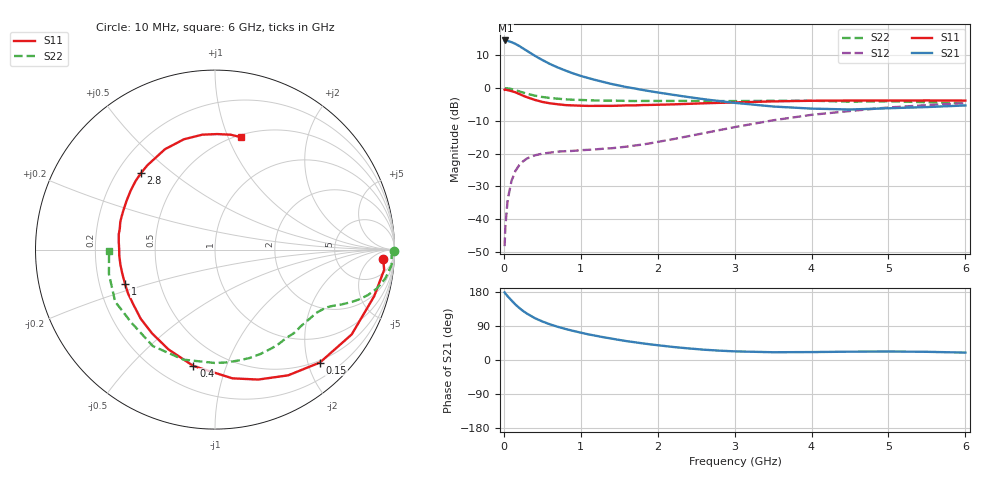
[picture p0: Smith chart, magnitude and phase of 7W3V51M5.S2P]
! Infineon Technologies  Discrete & RF Semiconductors
! BFS17W
! Si NPN RF Bipolar Junction Transistor in SOT323
! VCE = 3.5 V  IC = 1.5 mA
! Common Emitter S-Parameters:  August  1999
# GHz  S  MA  R  50
!  f  S11  S21  S12  S22
! GHz  MAG  ANG  MAG  ANG  MAG  ANG  MAG  ANG
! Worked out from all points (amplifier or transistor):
!   36 points, 10 MHz to 6 GHz, reference 50 ohm
!   highest |S21| = 14.5 dB at 20 MHz (marker M1)
!   |S21| within 3 dB of that: start of sweep to 288.9 MHz
!   unconditionally stable (mu >= 1): 905.5 MHz to end of sweep
!   at 250 MHz: K = 0.31, MSG = 17.2 dB, |S12| = -22.3 dB
!   at 1.4 GHz: K = 1.30, MAG = 6.5 dB, |S12| = -18.4 dB
!   at 6 GHz: K = 1.10, MAG = -2.2 dB, |S12| = -4.6 dB
!   S11 on the Smith chart (normalised r, x): 10 MHz: 18, -15; 150 MHz: 0.46, -2.21; 400 MHz: 0.34, -0.77; 1 GHz: 0.31, -0.17; 2.8 GHz: 0.30, +0.39; 6 GHz: 0.52, +1.11
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0.01  0.938 -3.2  5.265 178.3  0.0039 86.3  0.9998 -0.5
0.02  0.9493 -6.8  5.291 175.3  0.0078 91.6  0.9844 -2.0
0.05  0.9241 -16.3  5.204 168.1  0.0199 81.5  0.9877 -5.0
0.1  0.8964 -31.8  4.983 157.2  0.0386 71.8  0.9627 -9.6
0.15  0.8588 -47.1  4.702 146.5  0.0544 64.2  0.9266 -13.6
0.2  0.8105 -59.8  4.361 137.5  0.0668 58.6  0.8884 -16.6
0.25  0.7631 -71.6  4.001 129.5  0.0763 53.0  0.8503 -19.0
0.3  0.7238 -82.3  3.676 122.5  0.0843 49.1  0.8188 -20.8
0.4  0.6596 -100.5  3.108 110.8  0.0942 42.4  0.7656 -23.6
0.5  0.6136 -115.0  2.668 101.7  0.0999 38.8  0.7295 -25.4
0.6  0.5836 -127.0  2.316 94.1  0.1036 37.1  0.7037 -27.1
0.7  0.5653 -137.1  2.055 87.7  0.1073 36.4  0.6866 -29.0
0.8  0.5485 -145.7  1.845 82.0  0.109 36.1  0.6723 -30.9
1  0.5367 -159.1  1.527 72.2  0.1128 37.6  0.6572 -34.7
1.1  0.5334 -165.8  1.413 67.6  0.1144 38.8  0.65 -37.2
1.6  0.543 170.9  1.029 49.7  0.128 48.1  0.6346 -49.6
2.2  0.5628 151.1  0.787 34.4  0.1662 59.3  0.6343 -66.4
2.8  0.5934 134.0  0.631 24.7  0.228 63.6  0.632 -84.5
3.5  0.625 116.5  0.522 20.5  0.322 61.0  0.6377 -105.9
4.5  0.6442 96.3  0.47 22.0  0.4458 49.1  0.6186 -138.5
5.5  0.646 82.2  0.512 21.6  0.5475 36.2  0.6064 -167.0
6  0.6428 77.1  0.542 19.5  0.5861 30.0  0.5903 -179.5
